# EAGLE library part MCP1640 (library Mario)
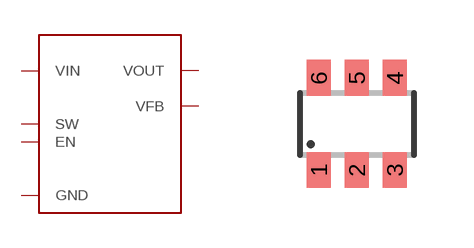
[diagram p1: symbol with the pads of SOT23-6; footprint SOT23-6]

Designator prefix -

## MCP1640  [SOT23-6]
1  SW
2  GND
3  EN
4  VFB
5  VOUT
6  VIN

## Footprint SOT23-6 (pad centres in mm)
smd 0.6 x 0.9: 1 -0.95,-1.15; 2 0,-1.15; 3 0.95,-1.15; 4 0.95,1.15; 5 0,1.15; 6 -0.95,1.15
